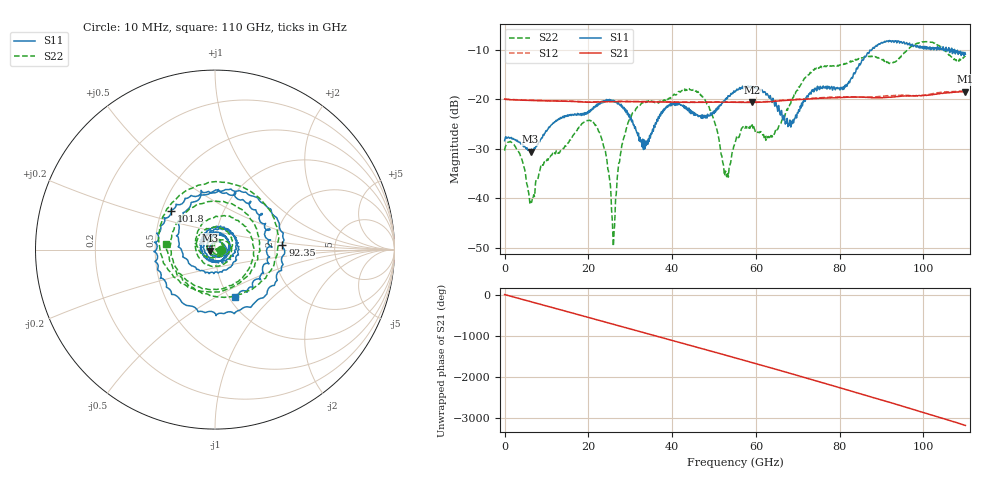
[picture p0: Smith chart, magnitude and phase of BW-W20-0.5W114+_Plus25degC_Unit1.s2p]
!Mini-Circuits Laboratory
!S-Parameters
!Model: BW-W20-0.5W114+
!Run / Lot / Date Code: QN2409253 /  / N/A
!Fixture:
!Network Analyzer: PNA-X N5242B - 423 4 ports (COM/DCOM);  Serial number: 74408
!Date: 3/8/2024 at 1:32:56 PM
!No.: Unit# 2 (U1  25C)
!Tested with:
# Hz  S  dB  R  50
!Frequency  S11 dB  S11 Deg  S21 dB  S21 Deg  S12 dB  S12 Deg  S22 dB  S22 Deg
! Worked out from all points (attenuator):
!   2208 points, 10 MHz to 110 GHz, reference 50 ohm
!   highest |S21| = -18.46 dB at 110 GHz (marker M1); lowest = -20.6 dB at 59.1 GHz (marker M2)
!   lowest |S11| = -30.6 dB at 6.2 GHz (marker M3), VSWR 1.06, Z = 47.2 - j0.483 ohm
!   |S11| at or under -10 dB: start of sweep to 87.69 GHz; 106.8 GHz to 107.4 GHz (582.1 MHz wide, 0.544 % of centre); 107.4 GHz to end of sweep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
!   |S22| runs from -49.6 to -8.4 dB; largest |S21 - S12| = 0.0054
!   S11 on the Smith chart (normalised r, x): 10 MHz: 1.08, -0.00; 92.35 GHz: 2.20, +0.13; 101.8 GHz: 0.56, +0.27; 110 GHz: 1.07, -0.61
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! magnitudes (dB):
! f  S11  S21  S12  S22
! 10 MHz  -28.4  -20.0  -19.9  -30.3
! 3.45 GHz  -28.6  -20.2  -20.1  -30.7
! 6.2 GHz  -30.6  -20.3  -20.2  -40.8
! 18.35 GHz  -23.2  -20.5  -20.5  -25.1
! 23.05 GHz  -20.6  -20.5  -20.5  -27.7
! 26 GHz  -20.3  -20.5  -20.4  -49.3
! 27.5 GHz  -21.1  -20.5  -20.4  -32.3
! 29.45 GHz  -22.9  -20.5  -20.4  -24.7
! 33.3 GHz  -28.2  -20.5  -20.5  -20.8
! 36.7 GHz  -23.6  -20.6  -20.5  -20.8
! 46.6 GHz  -23.4  -20.6  -20.6  -18.9
! 52.95 GHz  -19.8  -20.6  -20.5  -35.3
! 55.05 GHz  -18.4  -20.6  -20.5  -28.8
! 59.1 GHz  -17.6  -20.6  -20.6  -25.2
! 63.75 GHz  -20.3  -20.5  -20.4  -27.5
! 68.15 GHz  -24.2  -20.2  -20.1  -21.0
! 73.35 GHz  -18.1  -19.9  -19.8  -14.5
! 81.2 GHz  -17.2  -19.6  -19.5  -12.9
! 91.7 GHz  -8.4  -19.6  -19.3  -12.7
! 92.35 GHz  -8.5  -19.6  -19.3  -12.7
! 101.8 GHz  -9.7  -19.1  -18.9  -8.5
! 110 GHz  -10.9  -18.5  -18.3  -11.3
